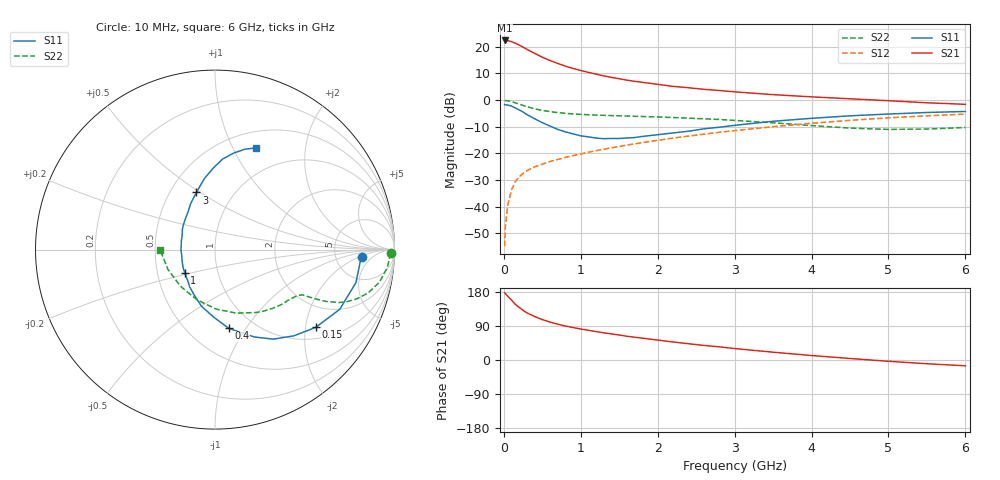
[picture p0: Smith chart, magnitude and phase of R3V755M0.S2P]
! SIEMENS Small Signal Semiconductors
! BFR181
! Si NPN RF Bipolar Junction Transistor in SOT23
! VCE = 0.75 V  IC = 5 mA
! Common Emitter S-Parameters:  May  1996
# GHz  S  MA  R  50
!  f  S11  S21  S12  S22
! GHz  MAG  ANG  MAG  ANG  MAG  ANG  MAG  ANG
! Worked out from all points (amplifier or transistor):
!   36 points, 10 MHz to 6 GHz, reference 50 ohm
!   highest |S21| = 22.4 dB at 10 MHz (marker M1)
!   |S21| within 3 dB of that: start of sweep to 279.6 MHz
!   unconditionally stable (mu >= 1): 815.9 MHz to 3.464 GHz
!   at 250 MHz: K = 0.47, MSG = 23.7 dB, |S12| = -27.6 dB
!   at 1.4 GHz: K = 1.13, MAG = 11.0 dB, |S12| = -17.9 dB
!   at 6 GHz: K = 0.93, MSG = 1.8 dB, |S12| = -5.3 dB
!   S11 on the Smith chart (normalised r, x): 10 MHz: 9.57, -2.26; 150 MHz: 1.31, -2.28; 400 MHz: 0.77, -0.84; 1 GHz: 0.69, -0.19; 3 GHz: 0.67, +0.48; 6 GHz: 0.68, +1.23
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0.01  0.82 -2.7  13.15 177.8  0.0018 94.9  0.9788 -1.2
0.02  0.8115 -5.1  13.13 175.2  0.0042 86.7  0.9748 -2.4
0.05  0.8066 -13.2  13.12 168.4  0.0105 81.0  0.9655 -5.9
0.1  0.7703 -25.6  12.48 157.8  0.0206 76.7  0.9343 -11.2
0.15  0.7087 -37.7  11.69 146.7  0.0293 70.6  0.8869 -15.8
0.2  0.6515 -47.5  10.78 138.6  0.0364 67.1  0.8375 -19.1
0.25  0.5948 -57.0  9.833 131.1  0.0419 63.6  0.7931 -21.4
0.3  0.5336 -65.8  8.968 124.4  0.047 62.4  0.7522 -23.1
0.4  0.4455 -80.1  7.529 114.7  0.0557 59.3  0.6839 -25.0
0.5  0.3752 -91.3  6.368 106.6  0.0624 59.0  0.6366 -25.9
0.6  0.3252 -103.2  5.537 100.2  0.0702 58.7  0.6055 -26.4
0.7  0.2808 -113.9  4.879 94.5  0.0764 59.2  0.5809 -26.8
0.8  0.2523 -123.7  4.333 89.7  0.0836 59.4  0.5634 -27.1
1  0.2127 -142.6  3.584 81.8  0.0968 60.5  0.5381 -28.1
1.1  0.2032 -151.4  3.309 78.4  0.1048 60.8  0.5294 -28.9
1.6  0.194 164.9  2.36 62.7  0.1424 61.1  0.5008 -33.8
2.2  0.2407 132.8  1.806 47.5  0.1929 59.4  0.4696 -42.4
3  0.3347 108.1  1.425 30.2  0.2663 54.0  0.4146 -57.8
3.5  0.3994 98.6  1.262 20.6  0.316 49.4  0.3734 -71.5
4.5  0.5052 85.3  1.055 4.0  0.4158 37.9  0.2971 -109.8
5.5  0.5834 73.5  0.888 -9.9  0.5059 24.6  0.2848 -157.3
6  0.6099 68.2  0.83 -15.3  0.5437 17.3  0.3048 -179.6
